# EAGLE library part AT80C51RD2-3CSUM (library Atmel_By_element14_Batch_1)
80C51 High Performance ROM 8-bit Microcontroller
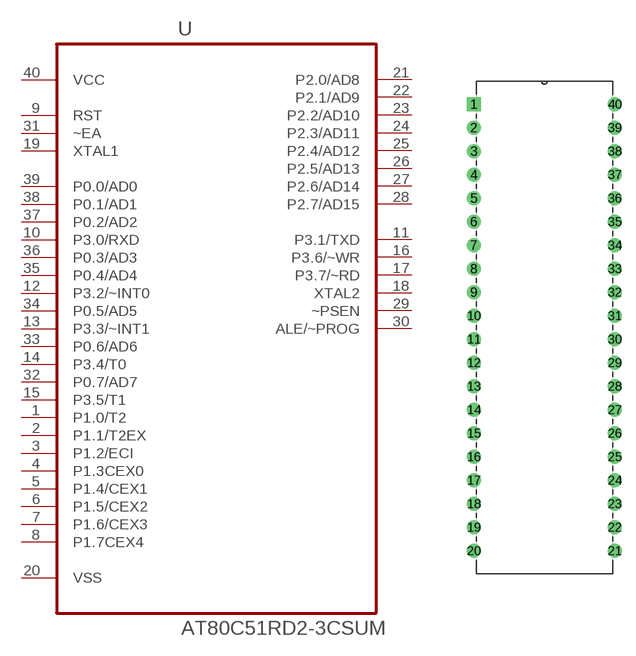
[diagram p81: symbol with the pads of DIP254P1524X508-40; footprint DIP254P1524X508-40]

Designator prefix U

## AT80C51RD2-3CSUM (MPN: AT80C51RD2-3CSUM; OC_FARNELL: 1699387; OC_NEWARK: 80P3686; PACKAGE: PDIL-40; SUPPLIER: Atmel)  [DIP254P1524X508-40]
1  P1.0/T2
2  P1.1/T2EX
3  P1.2/ECI
4  P1.3CEX0
5  P1.4/CEX1
6  P1.5/CEX2
7  P1.6/CEX3
8  P1.7CEX4
9  RST
10  P3.0/RXD  in
11  P3.1/TXD  out
12  P3.2/~INT0  in
13  P3.3/~INT1  in
14  P3.4/T0  in
15  P3.5/T1  in
16  P3.6/~WR  out
17  P3.7/~RD  out
18  XTAL2  out
19  XTAL1  in
20  VSS  pas
21  P2.0/AD8
22  P2.1/AD9
23  P2.2/AD10
24  P2.3/AD11
25  P2.4/AD12
26  P2.5/AD13
27  P2.6/AD14
28  P2.7/AD15
29  ~PSEN  out
30  ALE/~PROG  out
31  ~EA  in
32  P0.7/AD7
33  P0.6/AD6
34  P0.5/AD5
35  P0.4/AD4
36  P0.3/AD3
37  P0.2/AD2
38  P0.1/AD1
39  P0.0/AD0
40  VCC  pwr

## Footprint DIP254P1524X508-40 (pad centres in mm)
drill 0.991 square: 1 -15.24,48.26
drill 0.991: 2 -15.24,45.72; 3 -15.24,43.18; 4 -15.24,40.64; 5 -15.24,38.1; 6 -15.24,35.56; 7 -15.24,33.02; 8 -15.24,30.48; 9 -15.24,27.94; 10 -15.24,25.4; 11 -15.24,22.86; 12 -15.24,20.32; 13 -15.24,17.78; 14 -15.24,15.24; 15 -15.24,12.7; 16 -15.24,10.16; 17 -15.24,7.62; 18 -15.24,5.08; 19 -15.24,2.54; 20 -15.24,0; 21 0,0; 22 0,2.54; 23 0,5.08; 24 0,7.62; 25 0,10.16; 26 0,12.7; 27 0,15.24; 28 0,17.78; 29 0,20.32; 30 0,22.86; 31 0,25.4; 32 0,27.94; 33 0,30.48; 34 0,33.02; 35 0,35.56; 36 0,38.1; 37 0,40.64; 38 0,43.18; 39 0,45.72; 40 0,48.26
